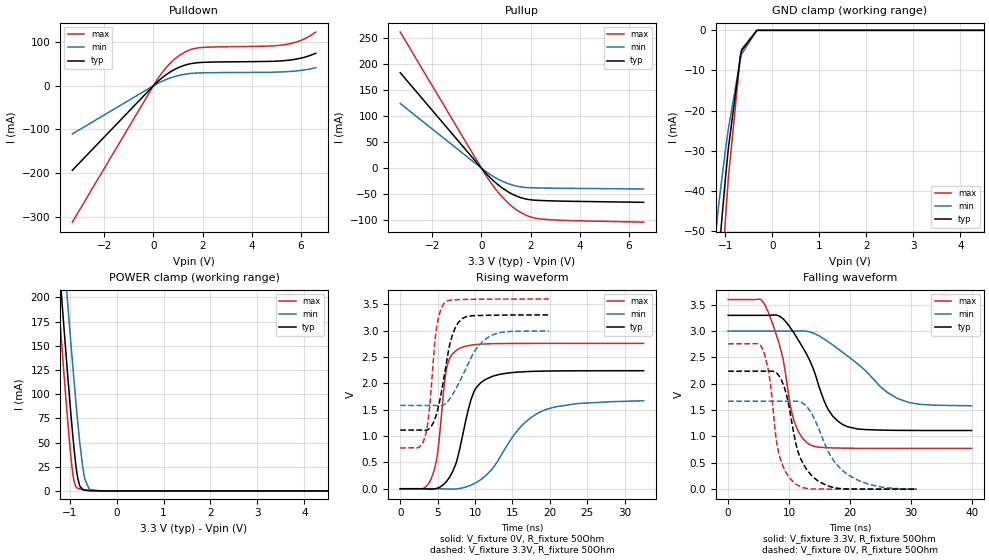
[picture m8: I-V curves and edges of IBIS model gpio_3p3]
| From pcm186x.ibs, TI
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|   gpio_3p3 Model
[Model]   gpio_3p3
Model_type   I/O
Polarity   Non-Inverting
Enable   Active-High
Vinl = 0.99
Vinh = 2.31
Vmeas = 1.65
Vref = 0
Cref = 2pF
Rref = 50
|   typ   min   max
|   (nom PVT)   (fast PVT)   (slow PVT)
C_comp   7.461e-12   7.393e-12   7.543e-12
[Model spec]
|subparameter
Vinl   0.99   0.9   1.08
Vinh   2.31   2.1   2.52
| Where nom  PVT is Nominal Process, 3.3V, 27C
|   Fast PVT is Strong Process,  3.6V, -40C
|   Slow PVT is Weak Process,   3V, 125C
[Voltage Range]   3.3   3   3.6
|Junction Temperature
[Temperature Range]   27   125   -40
[Pullup Reference]   3.3   3   3.6
[Pulldown Reference]   0   0   0
[Power Clamp Reference]   3.3   3   3.6
[GND Clamp Reference]   0   0   0
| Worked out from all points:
|   slope of the pulldown table from 0 to 0.495 V, typ, clamps not added: 20.3 ohm
|   slope of the pullup table from 0 to 0.495 V, typ, clamps not added: 20.3 ohm
|   POWER clamp passes 1 mA (typ) near -0.68 V on its own axis
|   falling waveform, V_fixture 3.3V, R_fixture 50Ohm: 20-80 % time 4.9ns typ, 8.42ns min, 3.1ns max; typ from 3.3 V to 1.11 V
|   rising waveform, V_fixture 0V, R_fixture 50Ohm: 20-80 % time 2.36ns typ, 5.35ns min, 1.25ns max; typ from 0 V to 2.24 V
|   rising waveform, V_fixture 3.3V, R_fixture 50Ohm: 20-80 % time 1.77ns typ, 3.17ns min, 1.07ns max; typ from 1.11 V to 3.3 V
|   falling waveform, V_fixture 0V, R_fixture 50Ohm: 20-80 % time 2.92ns typ, 4.86ns min, 1.98ns max; typ from 2.24 V to 0 V
[Pulldown]
|   Voltage   I(typ)   I(min)   I(max)
-3.3V     -193.6mA   -110.4mA   -312.3mA
114mV     6.395mA    3.598mA    10.54mA
471.9mV   23.47mA    13.24mA    38.45mA
858mV     37.16mA    20.93mA    60.71mA
1.251V    46.52mA    26.04mA    76.12mA
1.647V    51.7mA     28.64mA    84.9mA
2.043V    53.54mA    29.53mA    87.78mA
4.809V    55.69mA    30.84mA    90.87mA
5.308V    57.27mA    31.73mA    93.6mA
5.656V    59.52mA    32.99mA    97.49mA
6.084V    64.3mA     35.64mA    105.7mA
6.6V      74.25mA    41.12mA    122.7mA
[GND Clamp]
|   Voltage   I(typ)   I(min)   I(max)
-3.3V     -1.47A     -1.188A    -1.754A
-1.386V   -96.7mA    -70.76mA   -130.7mA
-1.154V   -58.38mA   -44.81mA   -77.05mA
-1.097V   -49.99mA   -39.02mA   -65.35mA
-1.005V   -37.66mA   -30.42mA   -48.23mA
-937.2mV  -29.45mA   -24.58mA   -36.91mA
-684mV    -6.73mA    -7.376mA   -6.767mA
-654mV    -5.034mA   -5.917mA   -4.726mA
-330mV    -4.08uA    -36.46uA   -660.2nA
6.6V      0A         0A         0A
[Pullup]
|   Voltage   I(typ)   I(min)   I(max)
-3.3V     183.6mA    124.3mA    261.7mA
158.4mV   -8.491mA   -5.726mA   -12.15mA
459mV     -22.87mA   -15.3mA    -32.96mA
699mV     -32.72mA   -21.72mA   -47.47mA
1.013V    -43.42mA   -28.47mA   -63.64mA
1.301V    -51.05mA   -33.04mA   -75.68mA
1.596V    -56.71mA   -36.09mA   -85.26mA
1.841V    -59.75mA   -37.4mA    -91.1mA
2.406V    -62.27mA   -38.2mA    -97.69mA
3.63V     -63.8mA    -38.91mA   -101mA
6.6V      -65.79mA   -40.15mA   -104mA
[POWER Clamp]
|   Voltage   I(typ)   I(min)   I(max)
-3.3V     1.681A     1.717A     1.676A
-1.27V    266.2mA    339.1mA    220.3mA
-1.136V   179.5mA    253.7mA    132.2mA
-1.08V    144.2mA    218.5mA    96.67mA
-1.018V   106.3mA    180.3mA    59.64mA
-934.8mV  59.44mA    131.1mA    19.28mA
-902.4mV  43.04mA    112.6mA    9.675mA
-825mV    13.11mA    70.88mA    2.759mA
-778.8mV  4.734mA    48.61mA    1.97mA
-690mV    1.091mA    16.09mA    1.001mA
-576mV    306.2uA    1.518mA    243.7uA
6.6V      0A         0A         0A
[Ramp]
R_load = 50
|   typ   min   max
dV/dt_r   1.34403/2.34396e-09   1.00197/5.30217e-09   1.65532/1.24688e-09
dV/dt_f   1.31203/4.89424e-09   0.850773/8.39678e-09   1.69538/3.08885e-09
[Falling Waveform]
V_fixture = 3.3V
V_fixture_min = 3V
V_fixture_max = 3.6V
R_fixture = 50Ohm
|   Time   V(typ)   V(min)   V(max)
0s        3.3V       3V         3.6V
5.995ns   3.3V       3V         3.509V
8.845ns   3.251V     3V         2.556V
10.22ns   3.065V     3V         1.587V
10.86ns   2.954V     3V         1.282V
13.26ns   2.479V     2.991V     857.5mV
16.4ns    1.519V     2.801V     786.6mV
19.57ns   1.187V     2.531V     777.6mV
27.86ns   1.117V     1.72V      774.7mV
39.98ns   1.113V     1.582V     774.3mV
[Rising Waveform]
V_fixture = 0V
V_fixture_min = 0V
V_fixture_max = 0V
R_fixture = 50Ohm
|   Time   V(typ)   V(min)   V(max)
0s        1.054nV    32.74nV    682.2pV
4.135ns   -8.348mV   -9.545uV   187.6mV
5.03ns    13.04mV    555.3uV    718.7mV
6.27ns    154.1mV    -5.504mV   2.333V
7.965ns   762.3mV    5.742mV    2.665V
9.825ns   1.831V     91.62mV    2.731V
12.31ns   2.132V     380mV      2.752V
15.81ns   2.214V     1.128V     2.758V
19.13ns   2.233V     1.483V     2.758V
32.55ns   2.24V      1.67V      2.759V
[Rising Waveform]
V_fixture = 3.3V
V_fixture_min = 3V
V_fixture_max = 3.6V
R_fixture = 50Ohm
|   Time   V(typ)   V(min)   V(max)
0s        1.113V     1.581V     774.3mV
2.415ns   1.113V     1.581V     776.4mV
3.255ns   1.108V     1.581V     958mV
3.885ns   1.143V     1.582V     1.488V
4.79ns    1.386V     1.579V     2.989V
5.96ns    2.207V     1.604V     3.534V
6.935ns   2.898V     1.772V     3.581V
8.28ns    3.228V     2.128V     3.591V
11.75ns   3.292V     2.873V     3.598V
19.88ns   3.299V     2.995V     3.6V
[Falling Waveform]
V_fixture = 0V
V_fixture_min = 0V
V_fixture_max = 0V
R_fixture = 50Ohm
|   Time   V(typ)   V(min)   V(max)
0s        2.24V      1.67V      2.759V
5.565ns   2.24V      1.67V      2.684V
6.785ns   2.241V     1.67V      2.129V
8.425ns   2.137V     1.67V      635.4mV
9.56ns    1.802V     1.67V      306.8mV
11.07ns   887.7mV    1.671V     101.3mV
13.84ns   244.2mV    1.41V      3.336mV
16.93ns   41.01mV    607.4mV    894.8uV
19.59ns   3.46mV     283.2mV    448.2uV
30.95ns   120.2uV    161.9uV    106.4uV
